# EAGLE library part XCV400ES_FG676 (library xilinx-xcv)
xcv400es_fg676 edit this description Auto generated by make-symbol-device-package-bsdl.ulp Rev. 26 Source: xcv400es_fg676.bsd
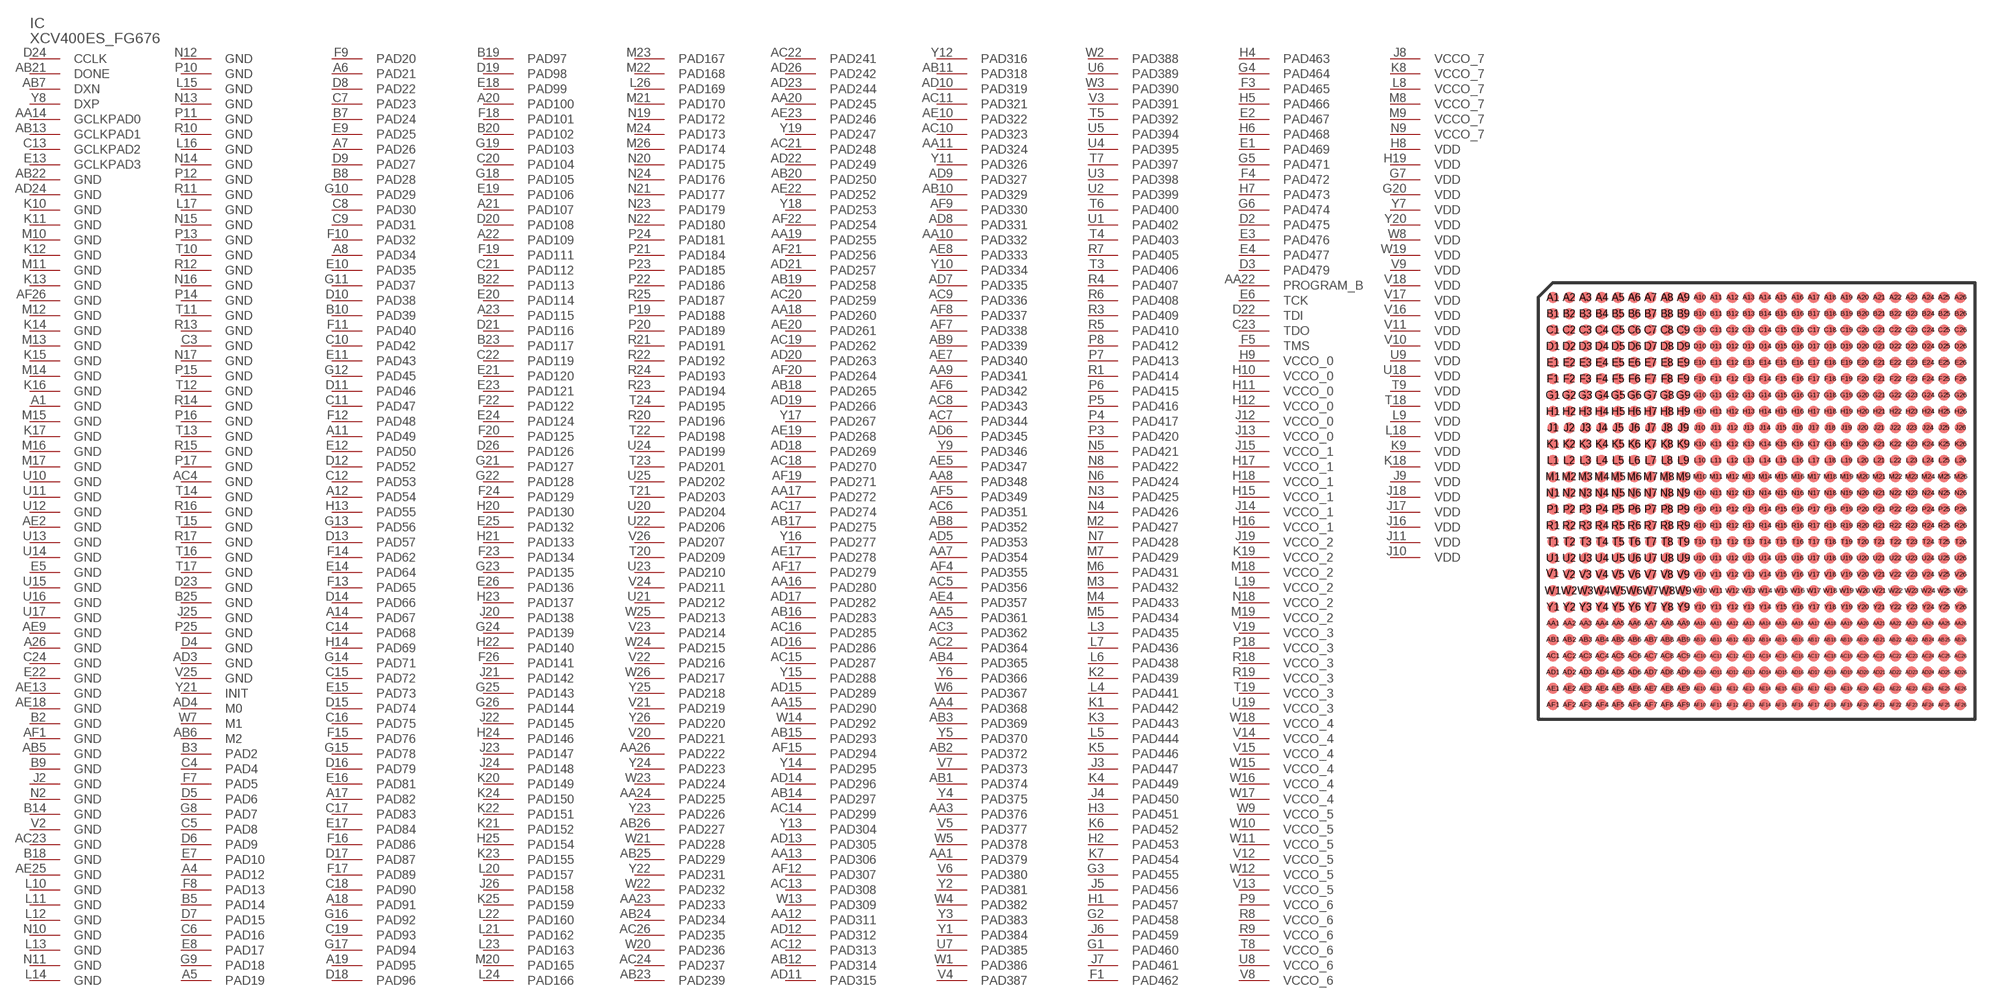
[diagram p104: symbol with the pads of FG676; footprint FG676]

Designator prefix IC

## XCV400ES_FG676 (OC_FARNELL: unknown; OC_NEWARK: unknown)  [FG676]
A1  GND  pwr
A4  PAD12
A5  PAD19
A6  PAD21
A7  PAD26
A8  PAD34
A11  PAD49
A12  PAD54
A14  PAD67
A17  PAD82
A18  PAD91
A19  PAD95
A20  PAD100
A21  PAD107
A22  PAD109
A23  PAD115
A26  GND  pwr
AA1  PAD379
AA3  PAD376
AA4  PAD368
AA5  PAD361
AA7  PAD354
AA8  PAD348
AA9  PAD341
AA10  PAD332
AA11  PAD324
AA12  PAD311
AA13  PAD306
AA14  GCLKPAD0  in
AA15  PAD290
AA16  PAD280
AA17  PAD272
AA18  PAD260
AA19  PAD255
AA20  PAD245
AA22  PROGRAM_B  in
AA23  PAD233
AA24  PAD225
AA26  PAD222
AB1  PAD374
AB2  PAD372
AB3  PAD369
AB4  PAD365
AB5  GND  pwr
AB6  M2  in
AB7  DXN  pas
AB8  PAD352
AB9  PAD339
AB10  PAD329
AB11  PAD318
AB12  PAD314
AB13  GCLKPAD1  in
AB14  PAD297
AB15  PAD293
AB16  PAD283
AB17  PAD275
AB18  PAD265
AB19  PAD258
AB20  PAD250
AB21  DONE
AB22  GND  pwr
AB23  PAD239
AB24  PAD234
AB25  PAD229
AB26  PAD227
AC2  PAD364
AC3  PAD362
AC4  GND  pwr
AC5  PAD356
AC6  PAD351
AC7  PAD344
AC8  PAD343
AC9  PAD336
AC10  PAD323
AC11  PAD321
AC12  PAD313
AC13  PAD308
AC14  PAD299
AC15  PAD287
AC16  PAD285
AC17  PAD274
AC18  PAD270
AC19  PAD262
AC20  PAD259
AC21  PAD248
AC22  PAD241
AC23  GND  pwr
AC24  PAD237
AC26  PAD235
AD3  GND  pwr
AD4  M0  in
AD5  PAD353
AD6  PAD345
AD7  PAD335
AD8  PAD331
AD9  PAD327
AD10  PAD319
AD11  PAD315
AD12  PAD312
AD13  PAD305
AD14  PAD296
AD15  PAD289
AD16  PAD286
AD17  PAD282
AD18  PAD269
AD19  PAD266
AD20  PAD263
AD21  PAD257
AD22  PAD249
AD23  PAD244
AD24  GND  pwr
AD26  PAD242
AE2  GND  pwr
AE4  PAD357
AE5  PAD347
AE7  PAD340
AE8  PAD333
AE9  GND  pwr
AE10  PAD322
AE13  GND  pwr
AE17  PAD278
AE18  GND  pwr
AE19  PAD268
AE20  PAD261
AE22  PAD252
AE23  PAD246
AE25  GND  pwr
AF1  GND  pwr
AF4  PAD355
AF5  PAD349
AF6  PAD342
AF7  PAD338
AF8  PAD337
AF9  PAD330
AF12  PAD307
AF15  PAD294
AF17  PAD279
AF19  PAD271
AF20  PAD264
AF21  PAD256
AF22  PAD254
AF26  GND  pwr
B2  GND  pwr
B3  PAD2
B5  PAD14
B7  PAD24
B8  PAD28
B9  GND  pwr
B10  PAD39
B14  GND  pwr
B18  GND  pwr
B19  PAD97
B20  PAD102
B22  PAD113
B23  PAD117
B25  GND  pwr
C3  GND  pwr
C4  PAD4
C5  PAD8
C6  PAD16
C7  PAD23
C8  PAD30
C9  PAD31
C10  PAD42
C11  PAD47
C12  PAD53
C13  GCLKPAD2  in
C14  PAD68
C15  PAD72
C16  PAD75
C17  PAD83
C18  PAD90
C19  PAD93
C20  PAD104
C21  PAD112
C22  PAD119
C23  TDO  out
C24  GND  pwr
D2  PAD475
D3  PAD479
D4  GND  pwr
D5  PAD6
D6  PAD9
D7  PAD15
D8  PAD22
D9  PAD27
D10  PAD38
D11  PAD46
D12  PAD52
D13  PAD57
D14  PAD66
D15  PAD74
D16  PAD79
D17  PAD87
D18  PAD96
D19  PAD98
D20  PAD108
D21  PAD116
D22  TDI  in
D23  GND  pwr
D24  CCLK
D26  PAD126
E1  PAD469
E2  PAD467
E3  PAD476
E4  PAD477
E5  GND  pwr
E6  TCK  in
E7  PAD10
E8  PAD17
E9  PAD25
E10  PAD35
E11  PAD43
E12  PAD50
E13  GCLKPAD3  in
E14  PAD64
E15  PAD73
E16  PAD81
E17  PAD84
E18  PAD99
E19  PAD106
E20  PAD114
E21  PAD120
E22  GND  pwr
E23  PAD121
E24  PAD124
E25  PAD132
E26  PAD136
F1  PAD462
F3  PAD465
F4  PAD472
F5  TMS  in
F7  PAD5
F8  PAD13
F9  PAD20
F10  PAD32
F11  PAD40
F12  PAD48
F13  PAD65
F14  PAD62
F15  PAD76
F16  PAD86
F17  PAD89
F18  PAD101
F19  PAD111
F20  PAD125
F22  PAD122
F23  PAD134
F24  PAD129
F26  PAD141
G1  PAD460
G2  PAD458
G3  PAD455
G4  PAD464
G5  PAD471
G6  PAD474
G7  VDD  pwr
G8  PAD7
G9  PAD18
G10  PAD29
G11  PAD37
G12  PAD45
G13  PAD56
G14  PAD71
G15  PAD78
G16  PAD92
G17  PAD94
G18  PAD105
G19  PAD103
G20  VDD  pwr
G21  PAD127
G22  PAD128
G23  PAD135
G24  PAD139
G25  PAD143
G26  PAD144
H1  PAD457
H2  PAD453
H3  PAD451
H4  PAD463
H5  PAD466
H6  PAD468
H7  PAD473
H8  VDD  pwr
H9  VCCO_0  pwr
H10  VCCO_0  pwr
H11  VCCO_0  pwr
H12  VCCO_0  pwr
H13  PAD55
H14  PAD69
H15  VCCO_1  pwr
H16  VCCO_1  pwr
H17  VCCO_1  pwr
H18  VCCO_1  pwr
H19  VDD  pwr
H20  PAD130
H21  PAD133
H22  PAD140
H23  PAD137
H24  PAD146
H25  PAD154
J2  GND  pwr
J3  PAD447
J4  PAD450
J5  PAD456
J6  PAD459
J7  PAD461
J8  VCCO_7  pwr
J9  VDD  pwr
J10  VDD  pwr
J11  VDD  pwr
J12  VCCO_0  pwr
J13  VCCO_0  pwr
J14  VCCO_1  pwr
J15  VCCO_1  pwr
J16  VDD  pwr
J17  VDD  pwr
J18  VDD  pwr
J19  VCCO_2  pwr
J20  PAD138
J21  PAD142
J22  PAD145
J23  PAD147
J24  PAD148
J25  GND  pwr
J26  PAD158
K1  PAD442
K2  PAD439
K3  PAD443
K4  PAD449
K5  PAD446
K6  PAD452
K7  PAD454
K8  VCCO_7  pwr
K9  VDD  pwr
K10  GND  pwr
K11  GND  pwr
K12  GND  pwr
K13  GND  pwr
K14  GND  pwr
K15  GND  pwr
K16  GND  pwr
K17  GND  pwr
K18  VDD  pwr
K19  VCCO_2  pwr
K20  PAD149
K21  PAD152
K22  PAD151
K23  PAD155
K24  PAD150
K25  PAD159
L3  PAD435
L4  PAD441
L5  PAD444
L6  PAD438
L7  PAD436
L8  VCCO_7  pwr
L9  VDD  pwr
L10  GND  pwr
L11  GND  pwr
L12  GND  pwr
L13  GND  pwr
L14  GND  pwr
L15  GND  pwr
L16  GND  pwr
L17  GND  pwr
L18  VDD  pwr
L19  VCCO_2  pwr
L20  PAD157
L21  PAD162
L22  PAD160
L23  PAD163
L24  PAD166
L26  PAD169
M2  PAD427
M3  PAD432
M4  PAD433
M5  PAD434
M6  PAD431
M7  PAD429
M8  VCCO_7  pwr
M9  VCCO_7  pwr
M10  GND  pwr
M11  GND  pwr
M12  GND  pwr
M13  GND  pwr
M14  GND  pwr
M15  GND  pwr
M16  GND  pwr
M17  GND  pwr
M18  VCCO_2  pwr
M19  VCCO_2  pwr
M20  PAD165
M21  PAD170
M22  PAD168
M23  PAD167
M24  PAD173
M26  PAD174
N2  GND  pwr
N3  PAD425
N4  PAD426
N5  PAD421
N6  PAD424
N7  PAD428
N8  PAD422
N9  VCCO_7  pwr
N10  GND  pwr
N11  GND  pwr
N12  GND  pwr
N13  GND  pwr
N14  GND  pwr
N15  GND  pwr
N16  GND  pwr
N17  GND  pwr
N18  VCCO_2  pwr
N19  PAD172
N20  PAD175
N21  PAD177
N22  PAD180
N23  PAD179
N24  PAD176
P3  PAD420
P4  PAD417
P5  PAD416
P6  PAD415
P7  PAD413
P8  PAD412
P9  VCCO_6  pwr
P10  GND  pwr
P11  GND  pwr
P12  GND  pwr
P13  GND  pwr
P14  GND  pwr
P15  GND  pwr
P16  GND  pwr
P17  GND  pwr
P18  VCCO_3  pwr
P19  PAD188
P20  PAD189
P21  PAD184
P22  PAD186
P23  PAD185
P24  PAD181
P25  GND  pwr
R1  PAD414
R3  PAD409
R4  PAD407
R5  PAD410
R6  PAD408
R7  PAD405
R8  VCCO_6  pwr
R9  VCCO_6  pwr
R10  GND  pwr
R11  GND  pwr
R12  GND  pwr
R13  GND  pwr
R14  GND  pwr
R15  GND  pwr
R16  GND  pwr
R17  GND  pwr
R18  VCCO_3  pwr
R19  VCCO_3  pwr
R20  PAD196
R21  PAD191
R22  PAD192
R23  PAD194
R24  PAD193
R25  PAD187
T3  PAD406
T4  PAD403
T5  PAD392
T6  PAD400
T7  PAD397
T8  VCCO_6  pwr
T9  VDD  pwr
T10  GND  pwr
T11  GND  pwr
T12  GND  pwr
T13  GND  pwr
T14  GND  pwr
T15  GND  pwr
T16  GND  pwr
T17  GND  pwr
T18  VDD  pwr
T19  VCCO_3  pwr
T20  PAD209
T21  PAD203
T22  PAD198
T23  PAD201
T24  PAD195
U1  PAD402
U2  PAD399
U3  PAD398
U4  PAD395
U5  PAD394
U6  PAD389
U7  PAD385
U8  VCCO_6  pwr
U9  VDD  pwr
U10  GND  pwr
U11  GND  pwr
U12  GND  pwr
U13  GND  pwr
U14  GND  pwr
U15  GND  pwr
U16  GND  pwr
U17  GND  pwr
U18  VDD  pwr
U19  VCCO_3  pwr
U20  PAD204
U21  PAD212
U22  PAD206
U23  PAD210
U24  PAD199
U25  PAD202
V2  GND  pwr
V3  PAD391
V4  PAD387
V5  PAD377
V6  PAD380
V7  PAD373
V8  VCCO_6  pwr
V9  VDD  pwr
V10  VDD  pwr
V11  VDD  pwr
V12  VCCO_5  pwr
V13  VCCO_5  pwr
V14  VCCO_4  pwr
V15  VCCO_4  pwr
V16  VDD  pwr
V17  VDD  pwr
V18  VDD  pwr
V19  VCCO_3  pwr
V20  PAD221
V21  PAD219
V22  PAD216
V23  PAD214
V24  PAD211
V25  GND  pwr
V26  PAD207
W1  PAD386
W2  PAD388
W3  PAD390
W4  PAD382
W5  PAD378
W6  PAD367
W7  M1  in
W8  VDD  pwr
W9  VCCO_5  pwr
W10  VCCO_5  pwr
W11  VCCO_5  pwr
W12  VCCO_5  pwr
W13  PAD309
W14  PAD292
W15  VCCO_4  pwr
W16  VCCO_4  pwr
W17  VCCO_4  pwr
W18  VCCO_4  pwr
W19  VDD  pwr
W20  PAD236
W21  PAD228
W22  PAD232
W23  PAD224
W24  PAD215
W25  PAD213
W26  PAD217
Y1  PAD384
Y2  PAD381
Y3  PAD383
Y4  PAD375
Y5  PAD370
Y6  PAD366
Y7  VDD  pwr
Y8  DXP  pas
Y9  PAD346
Y10  PAD334
Y11  PAD326
Y12  PAD316
Y13  PAD304
Y14  PAD295
Y15  PAD288
Y16  PAD277
Y17  PAD267
Y18  PAD253
Y19  PAD247
Y20  VDD  pwr
Y21  INIT
Y22  PAD231
Y23  PAD226
Y24  PAD223
Y25  PAD218
Y26  PAD220

## Footprint FG676 (pad centres in mm)
xcv400_fg676 edit this description Auto generated by make-symbol-device-package-bsdl.ulp Rev. 26 Source: xcv400_fg676.bsd
smd 0.7 x 0.7: A1 -12.5,12.5; A2 -11.5,12.5; A3 -10.5,12.5; A4 -9.5,12.5; A5 -8.5,12.5; A6 -7.5,12.5; A7 -6.5,12.5; A8 -5.5,12.5; A9 -4.5,12.5; A10 -3.5,12.5; A11 -2.5,12.5; A12 -1.5,12.5; A13 -0.5,12.5; A14 0.5,12.5; A15 1.5,12.5; A16 2.5,12.5; A17 3.5,12.5; A18 4.5,12.5; A19 5.5,12.5; A20 6.5,12.5; A21 7.5,12.5; A22 8.5,12.5; A23 9.5,12.5; A24 10.5,12.5; A25 11.5,12.5; A26 12.5,12.5; AA1 -12.5,-7.5; AA2 -11.5,-7.5; AA3 -10.5,-7.5; AA4 -9.5,-7.5; AA5 -8.5,-7.5; AA6 -7.5,-7.5; AA7 -6.5,-7.5; AA8 -5.5,-7.5; AA9 -4.5,-7.5; AA10 -3.5,-7.5; AA11 -2.5,-7.5; AA12 -1.5,-7.5; AA13 -0.5,-7.5; AA14 0.5,-7.5; AA15 1.5,-7.5; AA16 2.5,-7.5; AA17 3.5,-7.5; AA18 4.5,-7.5; AA19 5.5,-7.5; AA20 6.5,-7.5; AA21 7.5,-7.5; AA22 8.5,-7.5; AA23 9.5,-7.5; AA24 10.5,-7.5; AA25 11.5,-7.5; AA26 12.5,-7.5; AB1 -12.5,-8.5; AB2 -11.5,-8.5; AB3 -10.5,-8.5; AB4 -9.5,-8.5; AB5 -8.5,-8.5; AB6 -7.5,-8.5; AB7 -6.5,-8.5; AB8 -5.5,-8.5; AB9 -4.5,-8.5; AB10 -3.5,-8.5; AB11 -2.5,-8.5; AB12 -1.5,-8.5; AB13 -0.5,-8.5; AB14 0.5,-8.5; AB15 1.5,-8.5; AB16 2.5,-8.5; AB17 3.5,-8.5; AB18 4.5,-8.5; AB19 5.5,-8.5; AB20 6.5,-8.5; AB21 7.5,-8.5; AB22 8.5,-8.5; AB23 9.5,-8.5; AB24 10.5,-8.5; AB25 11.5,-8.5; AB26 12.5,-8.5; AC1 -12.5,-9.5; AC2 -11.5,-9.5; AC3 -10.5,-9.5; AC4 -9.5,-9.5; AC5 -8.5,-9.5; AC6 -7.5,-9.5; AC7 -6.5,-9.5; AC8 -5.5,-9.5; AC9 -4.5,-9.5; AC10 -3.5,-9.5; AC11 -2.5,-9.5; AC12 -1.5,-9.5; AC13 -0.5,-9.5; AC14 0.5,-9.5; AC15 1.5,-9.5; AC16 2.5,-9.5; AC17 3.5,-9.5; AC18 4.5,-9.5; AC19 5.5,-9.5; AC20 6.5,-9.5; AC21 7.5,-9.5; AC22 8.5,-9.5; AC23 9.5,-9.5; AC24 10.5,-9.5; AC25 11.5,-9.5; AC26 12.5,-9.5; AD1 -12.5,-10.5; AD2 -11.5,-10.5; AD3 -10.5,-10.5; AD4 -9.5,-10.5; AD5 -8.5,-10.5; AD6 -7.5,-10.5; AD7 -6.5,-10.5; AD8 -5.5,-10.5; AD9 -4.5,-10.5; AD10 -3.5,-10.5; AD11 -2.5,-10.5; AD12 -1.5,-10.5; AD13 -0.5,-10.5; AD14 0.5,-10.5; AD15 1.5,-10.5; AD16 2.5,-10.5; AD17 3.5,-10.5; AD18 4.5,-10.5; AD19 5.5,-10.5; AD20 6.5,-10.5; AD21 7.5,-10.5; AD22 8.5,-10.5; AD23 9.5,-10.5; AD24 10.5,-10.5; AD25 11.5,-10.5; AD26 12.5,-10.5; AE1 -12.5,-11.5; AE2 -11.5,-11.5; AE3 -10.5,-11.5; AE4 -9.5,-11.5; AE5 -8.5,-11.5; AE6 -7.5,-11.5; AE7 -6.5,-11.5; AE8 -5.5,-11.5; AE9 -4.5,-11.5; AE10 -3.5,-11.5; AE11 -2.5,-11.5; AE12 -1.5,-11.5; AE13 -0.5,-11.5; AE14 0.5,-11.5; AE15 1.5,-11.5; AE16 2.5,-11.5; AE17 3.5,-11.5; AE18 4.5,-11.5; AE19 5.5,-11.5; AE20 6.5,-11.5; AE21 7.5,-11.5; AE22 8.5,-11.5; AE23 9.5,-11.5; AE24 10.5,-11.5; AE25 11.5,-11.5; AE26 12.5,-11.5; AF1 -12.5,-12.5; AF2 -11.5,-12.5; AF3 -10.5,-12.5; AF4 -9.5,-12.5; AF5 -8.5,-12.5; AF6 -7.5,-12.5; AF7 -6.5,-12.5; AF8 -5.5,-12.5; AF9 -4.5,-12.5; AF10 -3.5,-12.5; AF11 -2.5,-12.5; AF12 -1.5,-12.5; AF13 -0.5,-12.5; AF14 0.5,-12.5; AF15 1.5,-12.5; AF16 2.5,-12.5; AF17 3.5,-12.5; AF18 4.5,-12.5; AF19 5.5,-12.5; AF20 6.5,-12.5; AF21 7.5,-12.5; AF22 8.5,-12.5; AF23 9.5,-12.5; AF24 10.5,-12.5; AF25 11.5,-12.5; AF26 12.5,-12.5; B1 -12.5,11.5; B2 -11.5,11.5; B3 -10.5,11.5; B4 -9.5,11.5; B5 -8.5,11.5; B6 -7.5,11.5; B7 -6.5,11.5; B8 -5.5,11.5; B9 -4.5,11.5; B10 -3.5,11.5; B11 -2.5,11.5; B12 -1.5,11.5; B13 -0.5,11.5; B14 0.5,11.5; B15 1.5,11.5; B16 2.5,11.5; B17 3.5,11.5; B18 4.5,11.5; B19 5.5,11.5; B20 6.5,11.5; B21 7.5,11.5; B22 8.5,11.5; B23 9.5,11.5; B24 10.5,11.5; B25 11.5,11.5; B26 12.5,11.5; C1 -12.5,10.5; C2 -11.5,10.5; C3 -10.5,10.5; C4 -9.5,10.5; C5 -8.5,10.5; C6 -7.5,10.5; C7 -6.5,10.5; C8 -5.5,10.5; C9 -4.5,10.5; C10 -3.5,10.5; C11 -2.5,10.5; C12 -1.5,10.5; C13 -0.5,10.5; C14 0.5,10.5; C15 1.5,10.5; C16 2.5,10.5; C17 3.5,10.5; C18 4.5,10.5; C19 5.5,10.5; C20 6.5,10.5; C21 7.5,10.5; C22 8.5,10.5; C23 9.5,10.5; C24 10.5,10.5; C25 11.5,10.5; C26 12.5,10.5; D1 -12.5,9.5; D2 -11.5,9.5; D3 -10.5,9.5; D4 -9.5,9.5; D5 -8.5,9.5; D6 -7.5,9.5; D7 -6.5,9.5; D8 -5.5,9.5; D9 -4.5,9.5; D10 -3.5,9.5; D11 -2.5,9.5; D12 -1.5,9.5; D13 -0.5,9.5; D14 0.5,9.5; D15 1.5,9.5; D16 2.5,9.5; D17 3.5,9.5; D18 4.5,9.5; D19 5.5,9.5; D20 6.5,9.5; D21 7.5,9.5; D22 8.5,9.5; D23 9.5,9.5; D24 10.5,9.5; D25 11.5,9.5; D26 12.5,9.5; E1 -12.5,8.5; E2 -11.5,8.5; E3 -10.5,8.5; E4 -9.5,8.5; E5 -8.5,8.5; E6 -7.5,8.5; E7 -6.5,8.5; E8 -5.5,8.5; E9 -4.5,8.5; E10 -3.5,8.5; E11 -2.5,8.5; E12 -1.5,8.5; E13 -0.5,8.5; E14 0.5,8.5; E15 1.5,8.5; E16 2.5,8.5; E17 3.5,8.5; E18 4.5,8.5; E19 5.5,8.5; E20 6.5,8.5; E21 7.5,8.5; E22 8.5,8.5; E23 9.5,8.5; E24 10.5,8.5; E25 11.5,8.5; E26 12.5,8.5; F1 -12.5,7.5; F2 -11.5,7.5; F3 -10.5,7.5; F4 -9.5,7.5; F5 -8.5,7.5; F6 -7.5,7.5; F7 -6.5,7.5; F8 -5.5,7.5; F9 -4.5,7.5; F10 -3.5,7.5; F11 -2.5,7.5; F12 -1.5,7.5; F13 -0.5,7.5; F14 0.5,7.5; F15 1.5,7.5; F16 2.5,7.5; F17 3.5,7.5; F18 4.5,7.5; F19 5.5,7.5; F20 6.5,7.5; F21 7.5,7.5; F22 8.5,7.5; F23 9.5,7.5; F24 10.5,7.5; F25 11.5,7.5; F26 12.5,7.5; G1 -12.5,6.5; G2 -11.5,6.5; G3 -10.5,6.5; G4 -9.5,6.5; G5 -8.5,6.5; G6 -7.5,6.5; G7 -6.5,6.5; G8 -5.5,6.5; G9 -4.5,6.5; G10 -3.5,6.5; G11 -2.5,6.5; G12 -1.5,6.5; G13 -0.5,6.5; G14 0.5,6.5; G15 1.5,6.5; G16 2.5,6.5; G17 3.5,6.5; G18 4.5,6.5; G19 5.5,6.5; G20 6.5,6.5; G21 7.5,6.5; G22 8.5,6.5; G23 9.5,6.5; G24 10.5,6.5; G25 11.5,6.5; G26 12.5,6.5; H1 -12.5,5.5; H2 -11.5,5.5; H3 -10.5,5.5; H4 -9.5,5.5; H5 -8.5,5.5; H6 -7.5,5.5; H7 -6.5,5.5; H8 -5.5,5.5; H9 -4.5,5.5; H10 -3.5,5.5; H11 -2.5,5.5; H12 -1.5,5.5; H13 -0.5,5.5; H14 0.5,5.5; H15 1.5,5.5; H16 2.5,5.5; H17 3.5,5.5; H18 4.5,5.5; H19 5.5,5.5; H20 6.5,5.5; H21 7.5,5.5; H22 8.5,5.5; H23 9.5,5.5; H24 10.5,5.5; H25 11.5,5.5; H26 12.5,5.5; J1 -12.5,4.5; J2 -11.5,4.5; J3 -10.5,4.5; J4 -9.5,4.5; J5 -8.5,4.5; J6 -7.5,4.5; J7 -6.5,4.5; J8 -5.5,4.5; J9 -4.5,4.5; J10 -3.5,4.5; J11 -2.5,4.5; J12 -1.5,4.5; J13 -0.5,4.5; J14 0.5,4.5; J15 1.5,4.5; J16 2.5,4.5; J17 3.5,4.5; J18 4.5,4.5; J19 5.5,4.5; J20 6.5,4.5; J21 7.5,4.5; J22 8.5,4.5; J23 9.5,4.5; J24 10.5,4.5; J25 11.5,4.5; J26 12.5,4.5; K1 -12.5,3.5; K2 -11.5,3.5; K3 -10.5,3.5; K4 -9.5,3.5; K5 -8.5,3.5; K6 -7.5,3.5; K7 -6.5,3.5; K8 -5.5,3.5; K9 -4.5,3.5; K10 -3.5,3.5; K11 -2.5,3.5; K12 -1.5,3.5; K13 -0.5,3.5; K14 0.5,3.5; K15 1.5,3.5; K16 2.5,3.5; K17 3.5,3.5; K18 4.5,3.5; K19 5.5,3.5; K20 6.5,3.5; K21 7.5,3.5; K22 8.5,3.5; K23 9.5,3.5; K24 10.5,3.5; K25 11.5,3.5; K26 12.5,3.5; L1 -12.5,2.5; L2 -11.5,2.5; L3 -10.5,2.5; L4 -9.5,2.5; L5 -8.5,2.5; L6 -7.5,2.5; L7 -6.5,2.5; L8 -5.5,2.5; L9 -4.5,2.5; L10 -3.5,2.5; L11 -2.5,2.5; L12 -1.5,2.5; L13 -0.5,2.5; L14 0.5,2.5; L15 1.5,2.5; L16 2.5,2.5; L17 3.5,2.5; L18 4.5,2.5; L19 5.5,2.5; L20 6.5,2.5; L21 7.5,2.5; L22 8.5,2.5; L23 9.5,2.5; L24 10.5,2.5; L25 11.5,2.5; L26 12.5,2.5; M1 -12.5,1.5; M2 -11.5,1.5; M3 -10.5,1.5; M4 -9.5,1.5; M5 -8.5,1.5; M6 -7.5,1.5; M7 -6.5,1.5; M8 -5.5,1.5; M9 -4.5,1.5; M10 -3.5,1.5; M11 -2.5,1.5; M12 -1.5,1.5; M13 -0.5,1.5; M14 0.5,1.5; M15 1.5,1.5; M16 2.5,1.5; M17 3.5,1.5; M18 4.5,1.5; M19 5.5,1.5; M20 6.5,1.5; M21 7.5,1.5; M22 8.5,1.5; M23 9.5,1.5; M24 10.5,1.5; M25 11.5,1.5; M26 12.5,1.5; N1 -12.5,0.5; N2 -11.5,0.5; N3 -10.5,0.5; N4 -9.5,0.5; N5 -8.5,0.5; N6 -7.5,0.5; N7 -6.5,0.5; N8 -5.5,0.5; N9 -4.5,0.5; N10 -3.5,0.5; N11 -2.5,0.5; N12 -1.5,0.5; N13 -0.5,0.5; N14 0.5,0.5; N15 1.5,0.5; N16 2.5,0.5; N17 3.5,0.5; N18 4.5,0.5; N19 5.5,0.5; N20 6.5,0.5; N21 7.5,0.5; N22 8.5,0.5; N23 9.5,0.5; N24 10.5,0.5; N25 11.5,0.5; N26 12.5,0.5; P1 -12.5,-0.5; P2 -11.5,-0.5; P3 -10.5,-0.5; P4 -9.5,-0.5; P5 -8.5,-0.5; P6 -7.5,-0.5; P7 -6.5,-0.5; P8 -5.5,-0.5; P9 -4.5,-0.5; P10 -3.5,-0.5; P11 -2.5,-0.5; P12 -1.5,-0.5; P13 -0.5,-0.5; P14 0.5,-0.5; P15 1.5,-0.5; P16 2.5,-0.5; P17 3.5,-0.5; P18 4.5,-0.5; P19 5.5,-0.5; P20 6.5,-0.5; P21 7.5,-0.5; P22 8.5,-0.5; P23 9.5,-0.5; P24 10.5,-0.5; P25 11.5,-0.5; P26 12.5,-0.5; R1 -12.5,-1.5; R2 -11.5,-1.5; R3 -10.5,-1.5; R4 -9.5,-1.5; R5 -8.5,-1.5; R6 -7.5,-1.5; R7 -6.5,-1.5; R8 -5.5,-1.5; R9 -4.5,-1.5; R10 -3.5,-1.5; R11 -2.5,-1.5; R12 -1.5,-1.5; R13 -0.5,-1.5; R14 0.5,-1.5; R15 1.5,-1.5; R16 2.5,-1.5; R17 3.5,-1.5; R18 4.5,-1.5; R19 5.5,-1.5; R20 6.5,-1.5; R21 7.5,-1.5; R22 8.5,-1.5; R23 9.5,-1.5; R24 10.5,-1.5; R25 11.5,-1.5; R26 12.5,-1.5; T1 -12.5,-2.5; T2 -11.5,-2.5; T3 -10.5,-2.5; T4 -9.5,-2.5; T5 -8.5,-2.5; T6 -7.5,-2.5; T7 -6.5,-2.5; T8 -5.5,-2.5; T9 -4.5,-2.5; T10 -3.5,-2.5; T11 -2.5,-2.5; T12 -1.5,-2.5; T13 -0.5,-2.5; T14 0.5,-2.5; T15 1.5,-2.5; T16 2.5,-2.5; T17 3.5,-2.5; T18 4.5,-2.5; T19 5.5,-2.5; T20 6.5,-2.5; T21 7.5,-2.5; T22 8.5,-2.5; T23 9.5,-2.5; T24 10.5,-2.5; T25 11.5,-2.5; T26 12.5,-2.5; U1 -12.5,-3.5; U2 -11.5,-3.5; U3 -10.5,-3.5; U4 -9.5,-3.5; U5 -8.5,-3.5; U6 -7.5,-3.5; U7 -6.5,-3.5; U8 -5.5,-3.5; U9 -4.5,-3.5; U10 -3.5,-3.5; U11 -2.5,-3.5; U12 -1.5,-3.5; U13 -0.5,-3.5; U14 0.5,-3.5; U15 1.5,-3.5; U16 2.5,-3.5; U17 3.5,-3.5; U18 4.5,-3.5; U19 5.5,-3.5; U20 6.5,-3.5; U21 7.5,-3.5; U22 8.5,-3.5; U23 9.5,-3.5; U24 10.5,-3.5; U25 11.5,-3.5; U26 12.5,-3.5; V1 -12.527,-4.431; V2 -11.5,-4.5; V3 -10.5,-4.5; V4 -9.5,-4.5; V5 -8.5,-4.5; V6 -7.5,-4.5; V7 -6.5,-4.5; V8 -5.5,-4.5; V9 -4.5,-4.5; V10 -3.5,-4.5; V11 -2.5,-4.5; V12 -1.5,-4.5; V13 -0.5,-4.5; V14 0.5,-4.5; V15 1.5,-4.5; V16 2.5,-4.5; V17 3.5,-4.5; V18 4.5,-4.5; V19 5.5,-4.5; V20 6.5,-4.5; V21 7.5,-4.5; V22 8.5,-4.5; V23 9.5,-4.5; V24 10.5,-4.5; V25 11.5,-4.5; V26 12.5,-4.5; W1 -12.5,-5.5; W2 -11.5,-5.5; W3 -10.5,-5.5; W4 -9.5,-5.5; W5 -8.5,-5.5; W6 -7.5,-5.5; W7 -6.5,-5.5; W8 -5.5,-5.5; W9 -4.5,-5.5; W10 -3.5,-5.5; W11 -2.5,-5.5; W12 -1.5,-5.5; W13 -0.5,-5.5; W14 0.5,-5.5; W15 1.5,-5.5; W16 2.5,-5.5; W17 3.5,-5.5; W18 4.5,-5.5; W19 5.5,-5.5; W20 6.5,-5.5; W21 7.5,-5.5; W22 8.5,-5.5; W23 9.5,-5.5; W24 10.5,-5.5; W25 11.5,-5.5; W26 12.5,-5.5; Y1 -12.5,-6.5; Y2 -11.5,-6.5; Y3 -10.5,-6.5; Y4 -9.5,-6.5; Y5 -8.5,-6.5; Y6 -7.5,-6.5; Y7 -6.5,-6.5; Y8 -5.5,-6.5; Y9 -4.5,-6.5; Y10 -3.5,-6.5; Y11 -2.5,-6.5; Y12 -1.5,-6.5; Y13 -0.5,-6.5; Y14 0.5,-6.5; Y15 1.5,-6.5; Y16 2.5,-6.5; Y17 3.5,-6.5; Y18 4.5,-6.5; Y19 5.5,-6.5; Y20 6.5,-6.5; Y21 7.5,-6.5; Y22 8.5,-6.5; Y23 9.5,-6.5; Y24 10.5,-6.5; Y25 11.5,-6.5; Y26 12.5,-6.5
